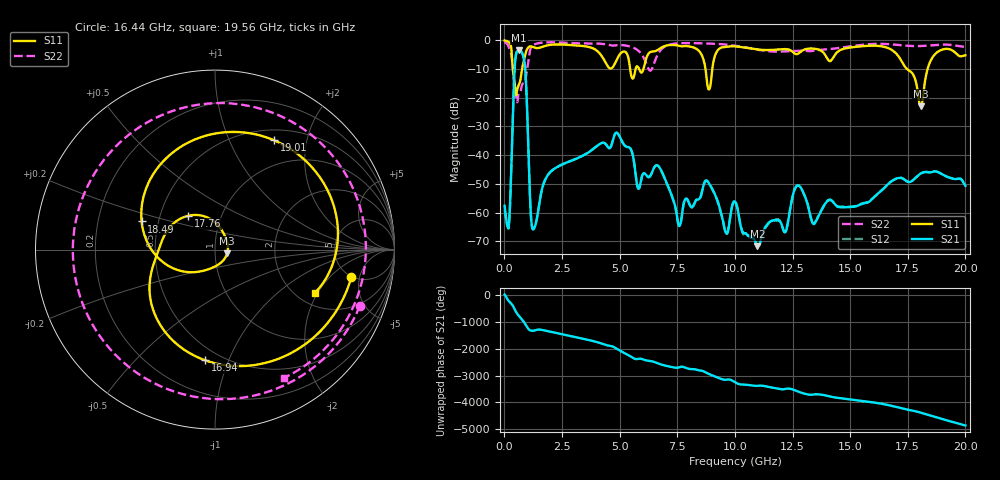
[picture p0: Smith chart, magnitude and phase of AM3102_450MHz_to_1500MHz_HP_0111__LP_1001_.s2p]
!Agilent Technologies,E8364B,MY43040894,A.07.50.67
!Agilent E8364B: A.07.50.67
!Date: Thursday, January 11, 2018 05:53:19
!Correction: S11(Full 2 Port(1,2))
!S21(Full 2 Port(1,2))
!S12(Full 2 Port(1,2))
!S22(Full 2 Port(1,2))
!S2P File: Measurements: S11, S21, S12, S22:
# Hz S  dB  R 50
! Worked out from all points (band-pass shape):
!   1601 points, 10 MHz to 20 GHz, reference 50 ohm
!   highest |S21| = -3.48 dB at 634.7 MHz (marker M1); lowest = -71.6 dB at 10.98 GHz (marker M2)
!   |S21| within 3 dB of the highest: 477.6 MHz to 845.5 MHz (367.8 MHz wide, 55.6 % of centre)
!   lowest |S11| = -23.0 dB at 18.06 GHz (marker M3), VSWR 1.15, Z = 57.2 - j2.43 ohm
!   |S11| at or under -10 dB: 368 MHz to 766.5 MHz (398.5 MHz wide, 70.3 % of centre); 8.725 GHz to 9.02 GHz (295 MHz wide, 3.33 % of centre); 17.47 GHz to 18.36 GHz (892.6 MHz wide, 4.98 % of centre)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
!   |S22| runs from -21.6 to -0.5 dB; largest |S21 - S12| = 0.0037
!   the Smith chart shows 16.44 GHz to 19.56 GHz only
!   S11 on the Smith chart (normalised r, x): 16.44 GHz: 4.91, -3.77; 16.94 GHz: 0.41, -0.83; 17.76 GHz: 0.70, +0.28; 18.49 GHz: 0.40, +0.16; 19.01 GHz: 0.63, +1.48; 19.56 GHz: 2.50, -1.90
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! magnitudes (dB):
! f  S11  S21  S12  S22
! 10 MHz  -0.1  -57.6  -58.9  -0.5
! 197.4 MHz  -0.7  -64.3  -64.2  -2.5
! 459.8 MHz  -16.0  -8.1  -8.1  -16.0
! 634.7 MHz  -15.3  -3.5  -3.5  -18.3
! 884.6 MHz  -5.8  -8.5  -8.5  -14.7
! 1.259 GHz  -2.4  -65.7  -65.7  -1.6
! 3.346 GHz  -1.9  -40.4  -40.4  -1.1
! 6.682 GHz  -3.2  -43.8  -43.8  -4.5
! 7.581 GHz  -2.0  -64.5  -64.6  -1.1
! 10.01 GHz  -2.1  -56.1  -56.0  -1.9
! 10.98 GHz  -3.2  -71.6  -71.4  -3.3
! 12.72 GHz  -4.8  -50.5  -50.6  -3.6
! 13.34 GHz  -2.9  -63.1  -62.8  -3.7
! 16.44 GHz  -2.2  -51.7  -51.7  -1.3
! 16.68 GHz  -2.8  -49.8  -49.8  -1.3
! 16.94 GHz  -4.2  -48.4  -48.4  -1.5
! 17.76 GHz  -12.4  -48.4  -48.4  -2.0
! 18.06 GHz  -23.0  -46.3  -46.4  -2.0
! 18.49 GHz  -7.2  -46.0  -45.9  -1.8
! 19.01 GHz  -3.2  -46.7  -46.8  -1.5
! 19.56 GHz  -4.3  -48.3  -48.3  -1.8
! 20 GHz  -5.2  -50.7  -50.7  -2.4
